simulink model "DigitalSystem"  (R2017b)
settings: Solver=VariableStepAuto  StartTime=0.0  StopTime=Tf  FixedStep=0.001  RelTol=1e-6
PostLoadFcn:
  | , if any(exist('dsrtsu_mdlpostloadfcn', 'file') == [2, 3, 6]), try dsrtsu_mdlpostloadfcn('Execute', bdroot); catch fprintf('Error in PostLoadFcn (dsrtsu_mdlpostloadfcn) for model "%s":\n %s\n', bdroot, lasterr); end, end,
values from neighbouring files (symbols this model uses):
  dd = dd(:)    [delaysModification.m]
  delta2 = 1/(delta2^2*(1+Kc^2))    [delayedModifiedSystemSimulation.m]    (also in delayedSystemSimulation.m; approximateLawsRLShunt.m; delayedModifiedSystemFRF.m; delayedSystemFRF.m)
  Kc = Kcv(nn)    [delayedModifiedSystemSimulation.m]    (also in delayedSystemSimulation.m; approximateLawsRLShunt.m; criticalDelays.m = Kc(:); delayedModifiedSystemFRF.m)
  q0 = 0    [delayedModifiedSystemSimulation.m]    (also in delayedSystemSimulation.m)
  tau = tauv(ii)    [delayedModifiedSystemSimulation.m]    (also in delayedSystemSimulation.m)
  Tf = 1e5    (= 100000)    [delayedModifiedSystemSimulation.m]    (also in delayedSystemSimulation.m)
  x0 = [0;0]    [delayedModifiedSystemSimulation.m]    (also in delayedSystemSimulation.m; homotopy.m = X(:,iter) + dx*dl)
  xd0 = 0    [delayedModifiedSystemSimulation.m]    (also in delayedSystemSimulation.m)
  zeta = zeta/sqrt(1+Kc^2)    [delayedModifiedSystemSimulation.m]    (also in delayedSystemSimulation.m; approximateLawsRLShunt.m; delayedModifiedSystemFRF.m; delayedSystemFRF.m)
undefined symbols (not defined in the file or in its folder): nd
libraries: simulink x1

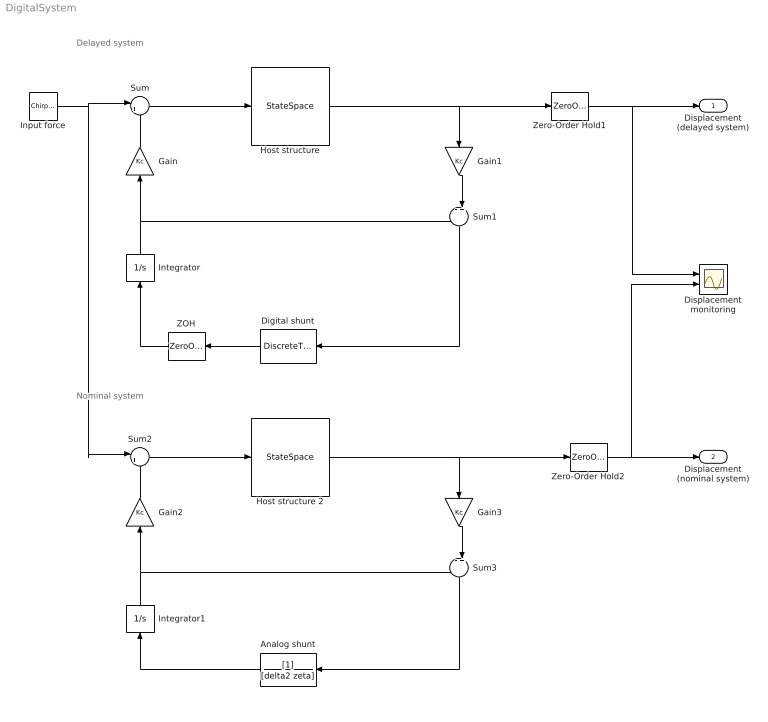
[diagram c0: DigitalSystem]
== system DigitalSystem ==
  note: Nominal system
  note: Delayed system
  Analog shunt : TransferFcn  Denominator=[delta2 zeta]
  Digital shunt : DiscreteTransferFcn  Numerator=nd  Denominator=dd  InitialStates=xd0  SampleTime=tau
  Displacement monitoring : Scope  NumInputPorts=2
  Gain{,1..3} (4 alike) : Gain  Gain=Kc
  Host structure : StateSpace  A=[0,1;-(1+Kc^2),0]  B=[0;1]  C=[1,0]  D=0  InitialCondition=x0
  Host structure 2 : StateSpace  A=[0,1;-(1+Kc^2),0]  B=[0;1]  C=[1,0]  D=0  InitialCondition=x0
  Input force : simulink/Sources/Chirp Signal  f1=w0/2/pi  T=Tf  f2=w1/2/pi
  Integrator : Integrator  InitialCondition=q0
  Integrator1 : Integrator  InitialCondition=q0
  Sum : Sum  Inputs=|++
  Sum1 : Sum  Inputs=-+|
  Sum2 : Sum  Inputs=|++
  Sum3 : Sum  Inputs=-+|
  ZOH : ZeroOrderHold  SampleTime=tau
  Zero-Order Hold1 : ZeroOrderHold  SampleTime=0.01
  Zero-Order Hold2 : ZeroOrderHold  SampleTime=0.01
  Displacement (delayed system) : Outport
  Displacement (nominal system) : Outport  Port=2
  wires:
  Input force/1 -> Sum2/1, Sum/1
  Sum1/1 -> Digital shunt/1
  Zero-Order Hold2/1 -> Displacement monitoring/2, Displacement (nominal system)/1
  Zero-Order Hold1/1 -> Displacement (delayed system)/1, Displacement monitoring/1
  Integrator/1 -> Sum1/1, Gain/1
  Host structure/1 -> Zero-Order Hold1/1, Gain1/1
  Gain3/1 -> Sum3/2
  Sum2/1 -> Host structure 2/1
  Integrator1/1 -> Sum3/1, Gain2/1
  Host structure 2/1 -> Zero-Order Hold2/1, Gain3/1
  Digital shunt/1 -> ZOH/1
  ZOH/1 -> Integrator/1
  Sum/1 -> Host structure/1
  Gain/1 -> Sum/2
  Gain1/1 -> Sum1/2
  Gain2/1 -> Sum2/2
  Sum3/1 -> Analog shunt/1
  Analog shunt/1 -> Integrator1/1
